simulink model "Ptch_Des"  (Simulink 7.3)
settings: Solver=ode45  StartTime=0.0  StopTime=100  RelTol=1e-3
undefined symbols (not defined in the file or in its folder): Ap, Bp, Cp, Dp

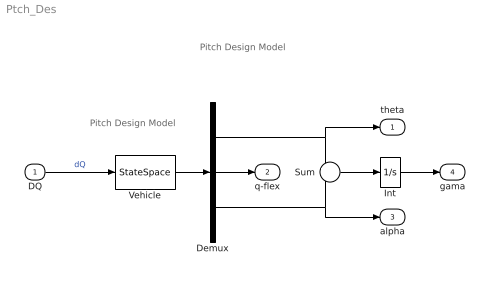
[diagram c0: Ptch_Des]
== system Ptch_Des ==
  note: Pitch Design Model
  note: Pitch Design Model
  DQ : Inport  OutDataType=sfix(16)  OutScaling=2^0
  Demux : Demux  Outputs=3
  Int : Integrator
  Sum : Sum  Inputs=+-  OutDataType=sfix(16)  OutScaling=2^0
  Vehicle : StateSpace  A=Ap  B=Bp  C=Cp  D=Dp
  theta : Outport  OutDataType=sfix(16)  OutScaling=2^0
  q-flex : Outport  Port=2  OutDataType=sfix(16)  OutScaling=2^0
  alpha : Outport  Port=3  OutDataType=sfix(16)  OutScaling=2^0
  gama : Outport  Port=4  OutDataType=sfix(16)  OutScaling=2^0
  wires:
  Vehicle/1 -> Demux/1
  Sum/1 -> Int/1
  Demux/1 -> theta/1, Sum/1
  Demux/2 -> q-flex/1
  Demux/3 -> alpha/1, Sum/2
  DQ/1 -> Vehicle/1  "dQ"
  Int/1 -> gama/1
